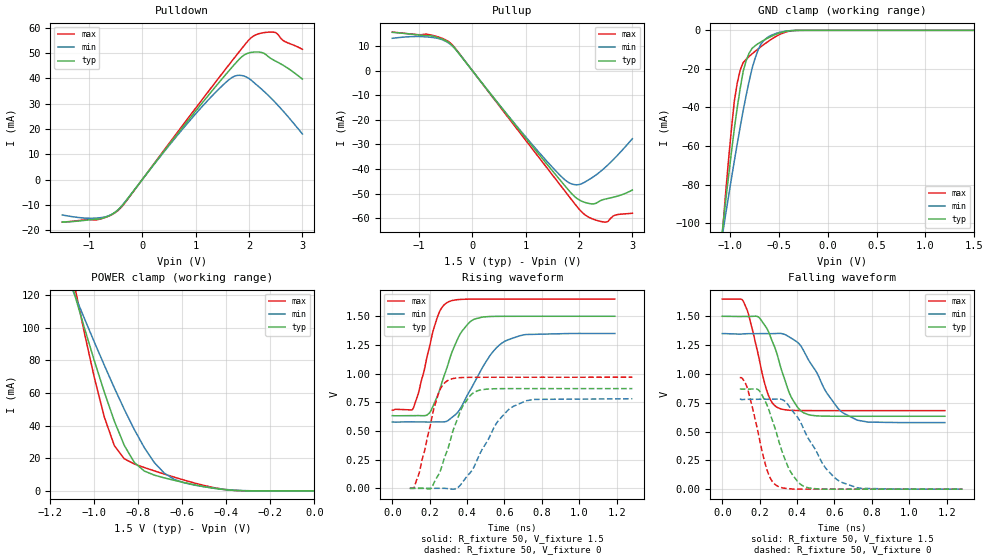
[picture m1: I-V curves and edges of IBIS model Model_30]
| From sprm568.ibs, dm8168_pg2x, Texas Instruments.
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| Model based on original model for BSHTLTCSCDVGPBFZ
|   Sub model SLOWEST_11MA_10PER_1P5
[model]   Model_30
|[Description]  [1.5V-3-STATE-X-SLOWEST:11MA, IND, 10%]
|   Slowest slew rate (SR[1:0] = "11"), 0.73 * RExt = 1.325 * Iout
|   (I[2:0] = "110"), 11mA nominal with Rext = 50R, ,Industrial
|   temperature range (-40C to 125C, 25C nominal),10% power supply
|   tolerance
|[Input Load]
|[Output Drive] SLOWEST:11MA
|Voltage   1.5V
|Mode   3-STATE
Model_type   3-state
Polarity   Non-Inverting
Enable   Active-Low
Cref =  15.0000pF
Rref =  100.0000M
Vref =  0V
Vmeas =  0.75
C_comp   1.5249p   1.4275p   1.6205p
[Model Spec]
[Temperature Range]   25   125   -40
[Voltage Range]   1.5   1.35   1.65
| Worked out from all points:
|   slope of the pulldown table from 0 to 0.225 V, typ, clamps not added: 36.2 ohm
|   slope of the pullup table from 0 to 0.225 V, typ, clamps not added: 36.1 ohm
|   GND clamp passes 1 mA (typ) near -0.47 V on its own axis
|   POWER clamp passes 1 mA (typ) near -0.42 V on its own axis
|   rising waveform, R_fixture 50, V_fixture 1.5: 20-80 % time 115ps typ, 164ps min, 87.5ps max; typ from 0.633 V to 1.5 V
|   rising waveform, R_fixture 50, V_fixture 0: 20-80 % time 109ps typ, 160ps min, 85.3ps max; typ from 0 V to 0.87 V
|   falling waveform, R_fixture 50, V_fixture 1.5: 20-80 % time 110ps typ, 168ps min, 84.6ps max; typ from 1.5 V to 0.632 V
|   falling waveform, R_fixture 50, V_fixture 0: 20-80 % time 110ps typ, 166ps min, 83.9ps max; typ from 0.869 V to 0 V
[POWER_clamp]
-1.5V     321.6mA    260.6mA    415.8mA
-1.091V   121.1mA    120.8mA    126.6mA
-1.076V   114.1mA    115.8mA    116.8mA
-1V       79.88mA    91.3mA     69.56mA
-954.5mV  60.58mA    77.05mA    45.34mA
-909.1mV  42.84mA    63.2mA     27.8mA
-818.2mV  17.47mA    37.6mA     16.51mA
-772.7mV  12.19mA    26.53mA    14.33mA
-681.8mV  7.985mA    10.89mA    10.33mA
-590.9mV  5.092mA    4.952mA    6.596mA
-363.6mV  298.9uA    465.6uA    298.1uA
0V        1.518nA    23.05nA    396.5pA
[Pulldown]
-1.5V     -16.86mA   -14.04mA   -16.9mA
-772.7mV  -15.51mA   -15.09mA   -15.55mA
-590.9mV  -14.04mA   -13.99mA   -14.12mA
-409.1mV  -11.11mA   -11mA      -11.35mA
954.5mV   25.91mA    24.89mA    26.98mA
1.455V    38.83mA    36.23mA    40.8mA
1.727V    45.55mA    40.89mA    48.2mA
2V        50.13mA    39.99mA    55.32mA
2.318V    49.42mA    34.17mA    58.25mA
2.5V      46.85mA    30.32mA    58.16mA
2.636V    45.27mA    27.17mA    55.07mA
3V        39.74mA    18.03mA    51.54mA
[Pullup]
-1.5V     15.55mA    13.13mA    15.65mA
-818.2mV  14.19mA    13.62mA    14.67mA
-409.1mV  10.85mA    10.66mA    11.17mA
1.227V    -33.46mA   -32.67mA   -34.7mA
1.682V    -45.43mA   -43.35mA   -47.47mA
1.864V    -50.03mA   -46.07mA   -52.55mA
2V        -52.51mA   -46.33mA   -56.27mA
2.182V    -53.99mA   -44.37mA   -59.58mA
2.409V    -52.78mA   -40.88mA   -61.31mA
2.545V    -51.96mA   -38.24mA   -61.26mA
2.682V    -51.26mA   -35.3mA    -58.71mA
3V        -48.54mA   -27.68mA   -57.97mA
[GND_clamp]
-1.5V     -310mA     -250.5mA   -402.4mA
-1.076V   -103.5mA   -106.1mA   -105.2mA
-1.045V   -89.74mA   -96.32mA   -85.93mA
-954.5mV  -51.19mA   -67.85mA   -36.85mA
-924.2mV  -40.06mA   -58.84mA   -27.27mA
-863.6mV  -21.23mA   -41.55mA   -16.73mA
-833.3mV  -15.79mA   -33.74mA   -15.03mA
-772.7mV  -9.342mA   -19.74mA   -12.19mA
-712.1mV  -6.927mA   -10.35mA   -9.702mA
-621.2mV  -4.26mA    -3.894mA   -6.224mA
-409.1mV  -336.9uA   -288.9uA   -618.6uA
1.5V      1.518nA    2.298uA    269.6pA
[Ramp]
dV/dt_f   0.694624/0.16817342n   0.619336/0.25049801n   0.775184/0.12345841n
dV/dt_r  0.7008416/0.17137846n 0.63054448/0.25047485n  0.7776068/0.12398346n
R_load = 50
[Rising Waveform]
R_fixture = 50
V_fixture = 1.5
V_fixture_min = 1.35
V_fixture_max = 1.65
0s        633.2mV    578.2mV    681.4mV
112.6ps   633.3mV    579.1mV    700mV
202.4ps   665.7mV    578.1mV    1.256V
251.4ps   848.6mV    578.8mV    1.535V
302.4ps   1.103V     595.9mV    1.627V
359.1ps   1.334V     682.8mV    1.646V
415.5ps   1.45V      852.5mV    1.649V
522.3ps   1.498V     1.157V     1.65V
598.6ps   1.5V       1.279V     1.65V
1.19ns    1.5V       1.35V      1.65V
[Rising Waveform]
R_fixture = 50
V_fixture = 0
V_fixture_min = 0
V_fixture_max = 0
93.89ps   0V         0V         0V
142.5ps   0V         0V         127.2mV
207ps     0V         0V         575mV
252.9ps   136.3mV    0V         849.8mV
299.2ps   353.6mV    -3.602mV   942.4mV
367.6ps   685.7mV    34.74mV    965.2mV
425.8ps   822.2mV    154.9mV    967.8mV
555.3ps   868.4mV    561.7mV    968.4mV
645.9ps   869.4mV    713.3mV    968.5mV
1.284ns   869.6mV    780.8mV    968.5mV
[Falling Waveform]
R_fixture = 50
V_fixture = 1.5
V_fixture_min = 1.35
V_fixture_max = 1.65
0s        1.5V       1.35V      1.649V
112.3ps   1.498V     1.347V     1.629V
199.3ps   1.485V     1.349V     1.114V
248.1ps   1.362V     1.349V     808.4mV
295.5ps   1.158V     1.351V     707.9mV
367.7ps   802.5mV    1.311V     683.9mV
458.4ps   647.4mV    1.129V     681.5mV
614.7ps   632.5mV    710.3mV    681.2mV
721.7ps   632.3mV    598.7mV    681.1mV
1.19ns    632.2mV    577.2mV    681.1mV
[Falling Waveform]
R_fixture = 50
V_fixture = 0
V_fixture_min = 0
V_fixture_max = 0
93.89ps   868.9mV    780mV      967.6mV
132.8ps   867.7mV    779.4mV    882.1mV
199.3ps   851.1mV    780mV      431.1mV
249.6ps   686.3mV    779.7mV    122mV
303.3ps   411.7mV    781.9mV    20.33mV
359.5ps   168.2mV    714.4mV    3.851mV
422.3ps   37.98mV    569mV      0V
548.1ps   0V         193.5mV    0V
642.5ps   0V         56.91mV    0V
1.284ns   0V         0V         0V
